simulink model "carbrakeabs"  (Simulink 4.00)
settings: Solver=ode45  StartTime=0.0  StopTime=Te  RelTol=1e-3
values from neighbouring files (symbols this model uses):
  c1 = 500    [bspbesch.m]    (also in bspofen.m = 921; carbrake.m = 0.857; ffwfback.m = [1 0]; kennwrt.m = 1)
  c2 = 921    [bspbesch.m]    (also in bspofen.m = 465; carbrake.m = 33.822; kennwrt.m = 1; schlupfsoll.m = 33.822)
  c3 = 465    [bspbesch.m]    (also in carbrake.m = 0.347; schlupfsoll.m = 0.347)
  dt = 0.1    [BatchTanks.m]    (also in carbrake.m = 0.01; fensterh.m = 0.005; kennwrt.m = 0.025; ljapst.m = (T(2)-T(1))/20)
  g = 9.81    [autobew.m]    (also in carbrake.m; drifter.m; ffwfback.m; ljapst.m)
  J = m*(ri*ri+ra*ra)/2    (= 24.217)    [carbrake.m]    (also in drehzr.m = 0.0013; fensterh.m = 1.3e-05; motor.m = 0.0013)
  m = 1000    [autobew.m]    (also in Bspreak.m = 10; carbrake.m = 250; drifter.m = 163.8; ffwfback.m = 0.3)
  omega0 = v0/r    (= 34.2090859332)    [carbrake.m]
  omegainf = 0    [carbrake.m]
  r = 0.406    [carbrake.m]    (also in ofenstb.m = [Ad(1,1)+Ad(2,2))
  v0 = 50/3.6    (= 13.8888888889)    [carbrake.m]
  vinf = 0.01    [carbrake.m]
  x0 = 5    [autobew.m]    (also in carbrake.m = 0; ffwfback.m = [phi0; phi0dot]; ljapst.m = [10/180*pi; 0]; motor.m = - inv(A)*B*12)
libraries: cstblocks x1

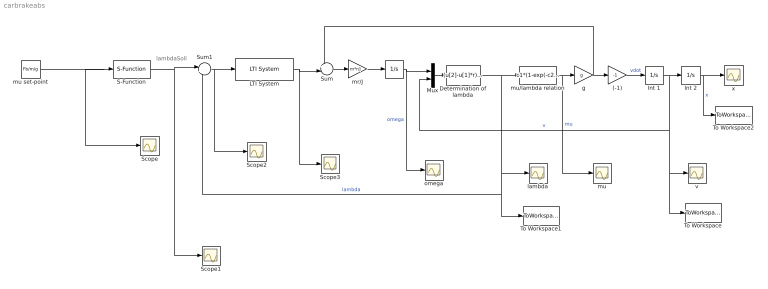
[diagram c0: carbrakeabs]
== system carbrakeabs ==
  note: lambdaSoll
  "  " : Integrator  ExternalReset=none  InitialConditionSource=internal  InitialCondition=omega0  LimitOutput=on  UpperSaturationLimit=inf  LowerSaturationLimit=omegainf  ShowSaturationPort=off  ShowStatePort=off  AbsoluteTolerance=auto
  (-1) : Gain  Gain=-1  Multiplication=Element-wise(K.*u)  SaturateOnIntegerOverflow=on
  Determination of lambda : Fcn  Expr=(u[2]-u[1]*r)/u[2]
  Int 1 : Integrator  ExternalReset=none  InitialConditionSource=internal  InitialCondition=v0  LimitOutput=on  UpperSaturationLimit=inf  LowerSaturationLimit=vinf  ShowSaturationPort=off  ShowStatePort=off  AbsoluteTolerance=auto
  Int 2 : Integrator  ExternalReset=none  InitialConditionSource=internal  InitialCondition=x0  LimitOutput=off  UpperSaturationLimit=inf  LowerSaturationLimit=0  ShowSaturationPort=off  ShowStatePort=off  AbsoluteTolerance=auto
  LTI System : cstblocks/LTI System  sys=300*tf([5 1],[5 0])  IC=0
  Mux : Mux  Inputs=2
  S-Function : S-Function  FunctionName=schlupfsoll  PortCounts=[]  SFunctionModules=''
  Scope{,1..3} (4 alike) : Scope
  Sum : Sum  Inputs=+-|  SaturateOnIntegerOverflow=on
  Sum1 : Sum  Inputs=|+-  SaturateOnIntegerOverflow=on
  To Workspace : ToWorkspace  VariableName=v  SampleTime=dt  SaveFormat=Array
  To Workspace1 : ToWorkspace  VariableName=lambda  SampleTime=dt  SaveFormat=Array
  To Workspace2 : ToWorkspace  VariableName=x  SampleTime=dt  SaveFormat=Array
  g : Gain  Gain=g  Multiplication=Element-wise(K.*u)  SaturateOnIntegerOverflow=on
  lambda : Scope
  mr/J : Gain  Gain=m*r/J  Multiplication=Element-wise(K.*u)  SaturateOnIntegerOverflow=on
  mu : Scope
  mu set-point : Constant  Value=Fb/m/g
  mu/lambda relation : Fcn  Expr=c1*(1-exp(-c2*u))-c3*u
  omega : Scope
  v : Scope
  x : Scope
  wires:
  mr/J/1 -> "  "/1
  "  "/1 -> Mux/1, omega/1  "omega"
  Mux/1 -> Determination of lambda/1
  Determination of lambda/1 -> mu/lambda relation/1, lambda/1, To Workspace1/1, Sum1/2  "lambda"
  mu/lambda relation/1 -> g/1, mu/1  "mu"
  Int 2/1 -> x/1, To Workspace2/1  "x"
  g/1 -> Sum/1, (-1)/1
  Int 1/1 -> Int 2/1, v/1, To Workspace/1, Mux/2  "v"
  (-1)/1 -> Int 1/1  "vdot"
  Sum/1 -> mr/J/1
  S-Function/1 -> Sum1/1, Scope1/1
  Sum1/1 -> LTI System/1, Scope2/1
  LTI System/1 -> Sum/2, Scope3/1
  mu set-point/1 -> S-Function/1, Scope/1
